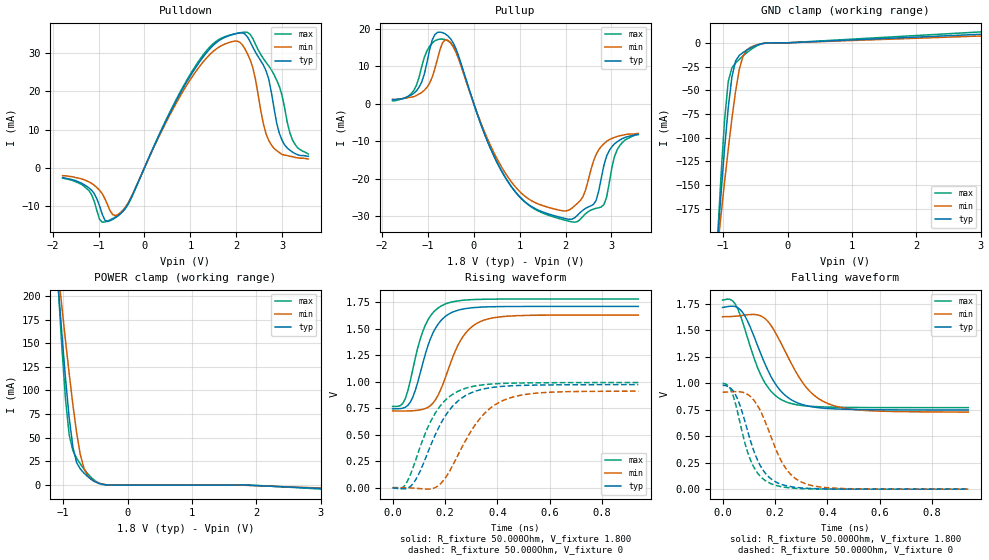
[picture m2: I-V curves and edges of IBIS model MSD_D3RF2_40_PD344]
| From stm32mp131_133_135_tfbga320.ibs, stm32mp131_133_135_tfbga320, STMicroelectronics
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[Model] MSD_D3RF2_40_PD344
Model_type   I/O
C_comp 2.313pF   2.232pF   2.432pF
Vinh = 1.150V
Vinl = 650.000mV
Vmeas = 900.000mV
Vref = 900.000mV
[Model Spec]
Vinh   1.150V   1.100V   1.200V
Vinl   650.000mV   600.000mV   700.000mV
Vmeas   900.000mV   850.000mV   950.000mV
Vref   900.000mV   850.000mV   950.000mV
[Temperature Range]   25.000   125.000   -40.000
[Voltage Range]   1.800V   1.700V   1.900V
[GND Clamp Reference]   0.00V   0.00V   0.00V
[Pulldown Reference]   0.00V   0.00V   0.00V
[POWER Clamp Reference]   1.800V   1.700V   1.900V
[Pullup Reference]   1.800V   1.700V   1.900V
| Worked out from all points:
|   slope of the pulldown table from 0 to 0.27 V, typ, clamps not added: 37.2 ohm
|   slope of the pullup table from 0 to 0.27 V, typ, clamps not added: 29.4 ohm
|   GND clamp passes 1 mA (typ) near -0.41 V on its own axis
|   POWER clamp passes 1 mA (typ) near -0.41 V on its own axis
|   rising waveform, R_fixture 50.000Ohm, V_fixture 1.800: 20-80 % time 78ps typ, 95.5ps min, 70.1ps max; typ from 0.743 V to 1.71 V
|   rising waveform, R_fixture 50.000Ohm, V_fixture 0: 20-80 % time 121ps typ, 139ps min, 110ps max; typ from -0.002 V to 0.971 V
|   falling waveform, R_fixture 50.000Ohm, V_fixture 1.800: 20-80 % time 110ps typ, 131ps min, 94.2ps max; typ from 1.71 V to 0.747 V
|   falling waveform, R_fixture 50.000Ohm, V_fixture 0: 20-80 % time 82.9ps typ, 99.5ps min, 71.1ps max; typ from 0.979 V to 0 V
[GND Clamp]
-1.785V   -901.2mA   -688.6mA   -1.21A
-1.094V   -214.7mA   -220.8mA   -215.3mA
-1.036V   -161.8mA   -183.6mA   -143.3mA
-978.8mV  -112.1mA   -147.2mA   -82.01mA
-921.2mV  -68.48mA   -112.4mA   -40.94mA
-863.6mV  -35.72mA   -79.61mA   -26.14mA
-806.1mV  -18.98mA   -50.62mA   -21.23mA
-748.5mV  -13.21mA   -27.8mA    -17.43mA
-690.9mV  -10.21mA   -13.8mA    -13.87mA
-575.8mV  -5.52mA    -4.739mA   -7.464mA
-345.4mV  -312.6uA   -378.8uA   -329uA
3.57V     10.68mA    8.508mA    13.66mA
[Power Clamp]
-1.77V    882.5mA    689.6mA    1.159A
-1.079V   212.4mA    226.4mA    212.1mA
-1.021V   160.9mA    189.3mA    146.7mA
-963.6mV  112.9mA    152.9mA    90.87mA
-906.1mV  71.13mA    117.8mA    52.88mA
-848.5mV  39.99mA    84.73mA    36.14mA
-790.9mV  23.76mA    55.38mA    28.45mA
-733.3mV  16.95mA    32.18mA    22.29mA
-618.2mV  8.932mA    9.702mA    11.91mA
-503mV    3.404mA    3.492mA    4.434mA
-330.3mV  151.6uA    319.4uA    178.5uA
3.585V    -5.406mA   -4.594mA   -6.496mA
[Pulldown]
-1.785V   -2.6mA     -2.1mA     -2.7mA
-1.209V   -5.3mA     -3.7mA     -6mA
-921.2mV  -12.19mA   -6.8mA     -14.28mA
-575.8mV  -12.61mA   -12.25mA   -12.48mA
1.152V    26.93mA    25.79mA    27.42mA
2.073V    35.35mA    32.95mA    35.37mA
2.361V    31.63mA    26.21mA    33.86mA
2.591V    26.91mA    11.5mA     28.61mA
2.764V    19.8mA     6mA        25.7mA
3.052V    6mA        3.3mA      15.8mA
3.224V    4.1mA      2.9mA      7.3mA
3.57V     3mA        2.3mA      3.6mA
[Pullup]
-1.77V    1.1mA      1.174mA    800uA
-1.309V   2.8mA      1.874mA    3.516mA
-1.021V   11mA       4.389mA    14.14mA
-848.5mV  18.49mA    9.339mA    16.82mA
-618.2mV  18.64mA    17.11mA    17.13mA
-387.9mV  14.68mA    13.71mA    14.14mA
763.6mV   -21.21mA   -19.96mA   -21.18mA
2.145V    -30.84mA   -27.84mA   -31.61mA
2.606V    -26.91mA   -15.4mA    -28.18mA
2.779V    -19.8mA    -11.41mA   -27.59mA
3.124V    -10.2mA    -8.753mA   -12.28mA
3.585V    -8.2mA     -7.926mA   -8.2mA
[Ramp]
R_load=50.000Ohm
dV/dt_r   579.930mV/99.500ps  543.329mV/118.500ps  600.120mV/90.500ps
dV/dt_f   579.930mV/97.000ps  543.329mV/116.000ps  600.120mV/83.500ps
[Rising waveform]
R_fixture=50.000Ohm
V_fixture=1.800
V_fixture_min=1.700
V_fixture_max=1.900
0s        743mV      723.1mV    765.4mV
39ps      749.2mV    722.2mV    794.1mV
68ps      806.8mV    723.7mV    1.01V
96ps      992.7mV    729.4mV    1.317V
125ps     1.259V     746.1mV    1.532V
163ps     1.5V       825.4mV    1.672V
202ps     1.615V     1.041V     1.732V
269ps     1.684V     1.425V     1.767V
355ps     1.704V     1.584V     1.776V
938ps     1.709V     1.627V     1.778V
[Rising waveform]
R_fixture=50.000Ohm
V_fixture=0
0s        -2.08mV    662.1uV    -2.63mV
39ps      -11.36mV   -403.6uV   1.187mV
77ps      33.35mV    -4.317mV   180.1mV
125ps     271.9mV    -13.82mV   512.6mV
163ps     499mV      341.6uV    703.5mV
202ps     678.6mV    93.51mV    825.4mV
259ps     835.1mV    352.5mV    919mV
345ps     929mV      684.3mV    969.1mV
441ps     958.8mV    840.3mV    984.2mV
938ps     971.1mV    909.7mV    990.9mV
[Falling waveform]
R_fixture=50.000Ohm
V_fixture=1.800
V_fixture_min=1.700
V_fixture_max=1.900
0s        1.714V     1.626V     1.783V
39ps      1.726V     1.629V     1.775V
77ps      1.666V     1.639V     1.572V
125ps     1.409V     1.647V     1.203V
154ps     1.227V     1.623V     1.036V
192ps     1.03V      1.517V     904.9mV
240ps     883.1mV    1.294V     825.8mV
326ps     784.6mV    941.4mV    783.4mV
422ps     757.9mV    789.4mV    773.4mV
938ps     746.9mV    727.3mV    768.9mV
[Falling waveform]
R_fixture=50.000Ohm
V_fixture=0
0s        979.2mV    913.7mV    996.9mV
20ps      970.4mV    916.8mV    979.6mV
39ps      931.7mV    919.5mV    893.1mV
68ps      779.6mV    918.1mV    610.8mV
106ps     460.3mV    874.7mV    278.5mV
144ps     220.7mV    741.7mV    121.1mV
183ps     100.9mV    506.8mV    53.8mV
250ps     28.54mV    167.7mV    14.26mV
336ps     6.536mV    36.82mV    2.737mV
938ps     8.307uV    18.37uV    -2.019uV
